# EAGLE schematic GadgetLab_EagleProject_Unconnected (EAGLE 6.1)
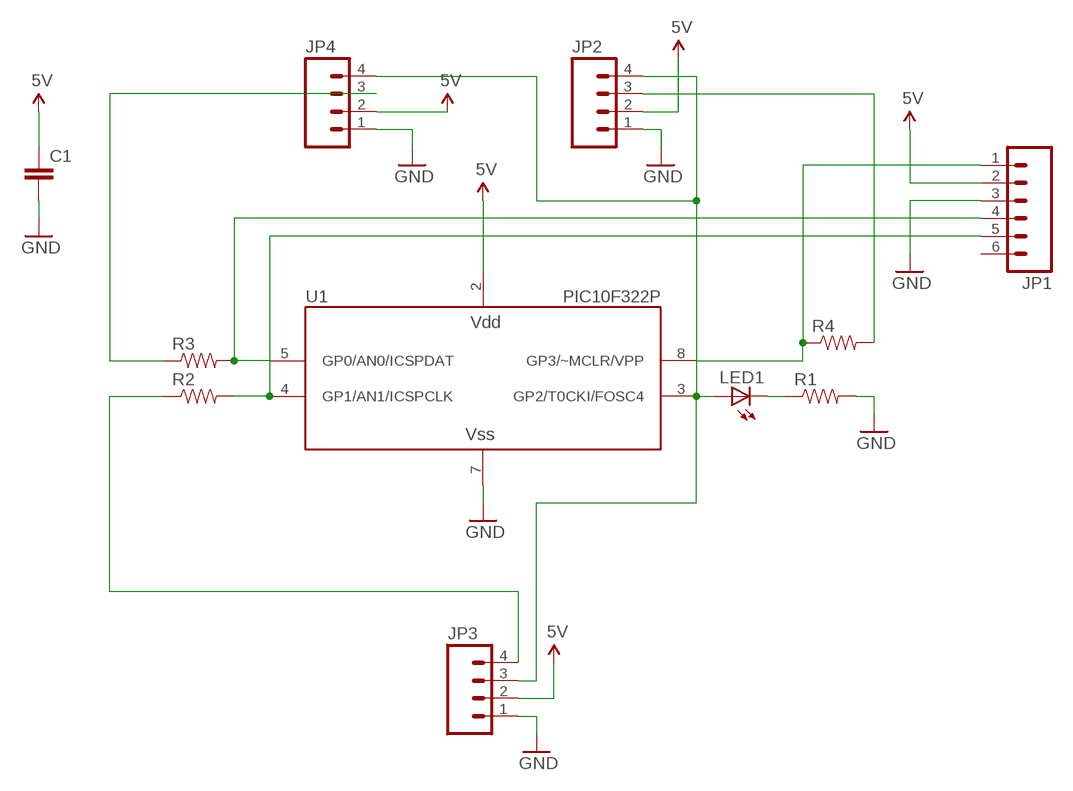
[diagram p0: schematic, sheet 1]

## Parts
C1  CAPPTH  [CAP-PTH-SMALL]
JP1  M06LOCK  [1X06_LOCK]
JP2  M04LOCK  [1X04_LOCK]
JP3  M04LOCK  [1X04_LOCK]
JP4  M04LOCK  [1X04_LOCK]
LED1  LED5MM  [LED5MM]
R1  RESISTORAXIAL-0.3  [AXIAL-0.3]
R2  RESISTORAXIAL-0.3  [AXIAL-0.3]
R3  RESISTORAXIAL-0.3  [AXIAL-0.3]
R4  RESISTORAXIAL-0.3  [AXIAL-0.3]
U1  PIC10F322P  [DIP-8]

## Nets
5V: C1.1 JP1.2 JP2.2 JP3.2 JP4.2 U1.2(VDD)
GND: C1.2 JP1.3 JP2.1 JP3.1 JP4.1 R1.P$2 U1.7(VSS)
N$1: JP2.4 JP3.3 JP4.4 LED1.A U1.3(GP2/T0CKI/FOSC4)
N$2: LED1.K(C) R1.P$1
N$3: JP1.1 R4.P$1 U1.8(GP3/~MCLR/VPP)
N$4: JP1.4 R3.P$2 U1.5(GP0/AN0/ICSPDAT)
N$5: JP1.5 R2.P$2 U1.4(GP1/AN1/ICSPCLK)
N$6: JP2.3 R4.P$2
N$8: JP4.3 R3.P$1
N$9: JP3.4 R2.P$1
Unconnected: JP1.6

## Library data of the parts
C1 = SparkFun:CAP: Capacitor
JP1 = SparkFun:M06: Header 6 Standard 6-pin 0.1" header. Use with straight break away headers (SKU : PRT-00116), right angle break away headers (PRT-00553), swiss pins (PRT-00743), machine pins (PRT-00117), and female headers (PRT-00115). Molex polarized connector foot print use with SKU : PRT-08094 with associated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
JP2-JP4 = SparkFun:M04: Header 4 Standard 4-pin 0.1" header. Use with straight break away headers (SKU : PRT-00116), right angle break away headers (PRT-00553), swiss pins (PRT-00743), machine pins (PRT-00117), and female headers (PRT-00115). Molex polarized connector foot print use with SKU : PRT-08231 with associated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
LED1 = SparkFun:LED: LEDs
R1-R4 = SparkFun:RESISTOR: Resistor
U1 = CindysStuff:PIC10F32*: Microchip PIC10F320 and 322 6-pin 8-bit Flash microcontroller 4 I/O, 2 8-bit timers, temperature sensor on PIC10F322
